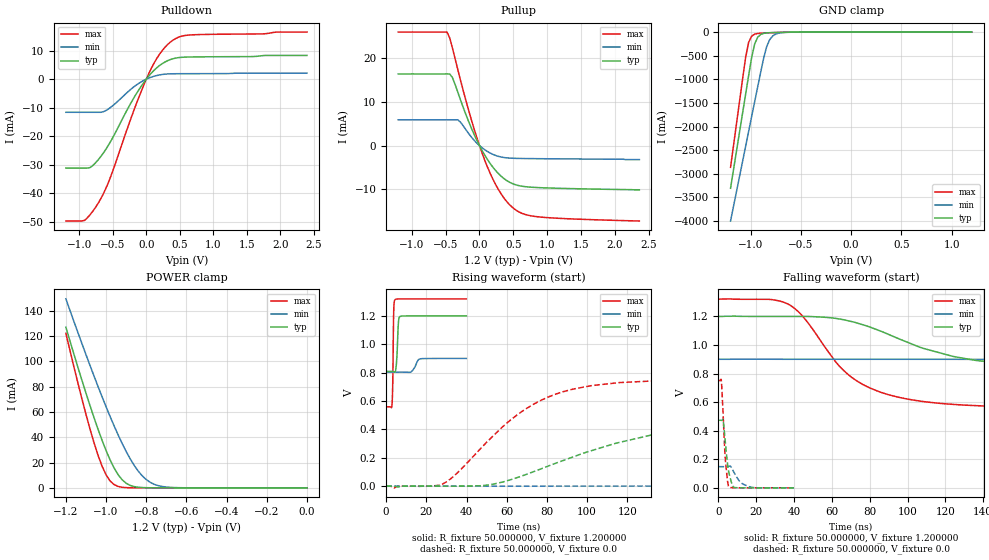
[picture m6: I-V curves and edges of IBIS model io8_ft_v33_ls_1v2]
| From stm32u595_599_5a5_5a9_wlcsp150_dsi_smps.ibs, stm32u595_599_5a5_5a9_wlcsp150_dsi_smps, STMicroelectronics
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|   Model io8_ft_v33_ls_1v2
[Model]  io8_ft_v33_ls_1v2
Model_type I/O
Polarity   Non-Inverting
Enable   Active-Low
Vinl =   0.360000V
Vinh =   0.840000V
Vmeas =  0.600000V
Cref =   50.000000pF
Rref =   100.000000M
Vref =   0.0V
C_comp   2.887200pF   2.816900pF   2.935200pF
[Temperature Range]   25.000000   0.140000k   -40.000000
[Pullup Reference]   1.200000V   0.900000V   1.320000V
[Pulldown Reference]   0.0V   0.0V   0.0V
[POWER Clamp Reference]   1.200000V   0.900000V   1.320000V
[GND Clamp Reference]   0.0V   0.0V   0.0V
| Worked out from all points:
|   slope of the pulldown table from 0 to 0.18 V, typ, clamps not added: 40.7 ohm
|   slope of the pullup table from 0 to 0.18 V, typ, clamps not added: 39.5 ohm
|   GND clamp passes 1 mA (typ) near -0.51 V on its own axis
|   POWER clamp passes 1 mA (typ) near -0.86 V on its own axis
|   rising waveform, R_fixture 50.000000, V_fixture 1.200000: 20-80 % time 752ps typ, 2.06ns min, 414ps max; typ from 0.809 V to 1.2 V
|   rising waveform, R_fixture 50.000000, V_fixture 0.0: 20-80 % time 67.6ns typ, 169ns min, 37.1ns max; typ from 0 V to 0.473 V
|   falling waveform, R_fixture 50.000000, V_fixture 1.200000: 20-80 % time 58.5ns typ, 150ns min, 31.6ns max; typ from 1.2 V to 0.809 V
|   falling waveform, R_fixture 50.000000, V_fixture 0.0: 20-80 % time 2.49ns typ, 4.76ns min, 1.84ns max; typ from 0.473 V to 0 V
[Pulldown]
|Voltage   I(typ)   I(min)   I(max)
-1.2V     -31.16mA   -11.61mA   -49.71mA
-920mV    -31.16mA   -11.61mA   -49.48mA
-840mV    -31mA      -11.61mA   -47.54mA
-720mV    -28.32mA   -11.61mA   -43.58mA
-560mV    -22.95mA   -10.37mA   -35.89mA
-200mV    -7.146mA   -2.964mA   -11.89mA
0V        0A         0A         0A
160mV     4.047mA    1.298mA    7.361mA
360mV     6.87mA     1.87mA     13mA
480mV     7.543mA    1.91mA     14.69mA
640mV     7.764mA    1.923mA    15.46mA
2.4V      8.316mA    2.102mA    16.52mA
[Pullup]
|Voltage   I(typ)   I(min)   I(max)
-1.2V     16.39mA    5.9mA      25.97mA
-480mV    16.39mA    5.9mA      25.97mA
-440mV    16.39mA    5.9mA      24.63mA
-400mV    15.57mA    5.9mA      22.35mA
-320mV    12.21mA    5.9mA      17.37mA
-120mV    3.997mA    1.962mA    5.905mA
80mV      -2.237mA   -962.6uA   -3.434mA
280mV     -6.404mA   -2.453mA   -10.06mA
520mV     -8.88mA    -2.901mA   -14.54mA
680mV     -9.389mA   -2.951mA   -15.76mA
920mV     -9.627mA   -2.991mA   -16.35mA
2.36V     -10.1mA    -3.2mA     -17.23mA
[GND_clamp]
|Voltage   I(typ)   I(min)   I(max)
-1.2V     -3.305A    -3.998A    -2.862A
-1.05V    -1.316A    -2.418A    -539.3mA
-1.02V    -921mA     -2.103A    -218.8mA
-990mV    -539.5mA   -1.788A    -87.43mA
-960mV    -252.1mA   -1.474A    -44.36mA
-930mV    -110.5mA   -1.16A     -30.32mA
-870mV    -28.03mA   -549.1mA   -21.09mA
-840mV    -18.43mA   -305.6mA   -18.27mA
-810mV    -13.9mA    -159.7mA   -15.73mA
-780mV    -11.23mA   -82.35mA   -13.37mA
-600mV    -2.976mA   -4.272mA   -3.058mA
1.2V      0A         14.74nA    0A
[POWER_clamp]
|Voltage   I(typ)   I(min)   I(max)
-1.2V     127mA      149.4mA    122.2mA
-1.12V    84.97mA    114mA      70.27mA
-1.06V    55.51mA    88.42mA    35.67mA
-1.02V    37.63mA    72.04mA    17.17mA
-1V       29.51mA    64.13mA    10.3mA
-960mV    15.69mA    48.99mA    2.571mA
-900mV    3.624mA    28.77mA    182.8uA
-840mV    490.7uA    13.24mA    11.35uA
-800mV    116.8uA    6.532mA    1.77uA
-740mV    13.2uA     1.723mA    109.1nA
-620mV    167.3nA    79.35uA    0A
0V        0A         17.84nA    0A
[Ramp]
| variable   typ   min   max
dV/dt_r  0.28374/67.55993n   88.87187m/0.16834u  0.45090/37.04554n
dV/dt_f  0.23463/58.41528n   57.86400m/0.14978u  0.45666/31.55745n
R_load = 50.000000
[Rising Waveform]
R_fixture= 50.000000
V_fixture= 1.200000
V_fixture_min= 0.900000
V_fixture_max= 1.320000
|time   V(typ)   V(min)   V(max)
0s        809mV      803.5mV    558.9mV
2.883ns   809.1mV    803.5mV    568.2mV
3.283ns   809mV      803.5mV    730.5mV
3.764ns   807.6mV    803.5mV    1.237V
4.404ns   804.5mV    803.5mV    1.314V
5.205ns   883.7mV    803.5mV    1.319V
6.166ns   1.164V     803.5mV    1.319V
6.807ns   1.195V     803.5mV    1.32V
16.98ns   1.2V       897.4mV    1.32V
39.88ns   1.2V       900mV      1.32V
[Rising Waveform]
R_fixture= 50.000000
V_fixture= 0.0
V_fixture_min= 0.0
V_fixture_max= 0.0
|time   V(typ)   V(min)   V(max)
0s        2.277nV    212.1nV    1.455nV
28.03ns   -71.47uV   -26.54uV   14mV
52.05ns   10.76mV    -20.37uV   337.8mV
74.07ns   105.7mV    7.748uV    583.1mV
92.09ns   201.2mV    73.5uV     680.8mV
118.1ns   315mV      425.6uV    731.4mV
168.2ns   427.6mV    6.838mV    749.9mV
244.2ns   467mV      48.53mV    751.6mV
452.5ns   472.9mV    134.9mV    751.5mV
997ns     472.9mV    148.2mV    751.6mV
[Falling Waveform]
R_fixture= 50.000000
V_fixture= 1.200000
V_fixture_min= 0.900000
V_fixture_max= 1.320000
|time   V(typ)   V(min)   V(max)
0s        1.2V       900mV      1.32V
36.04ns   1.2V       900mV      1.291V
44.04ns   1.2V       900mV      1.209V
64.06ns   1.182V     900mV      850.1mV
76.08ns   1.143V     900mV      725.6mV
98.1ns    1.029V     900mV      626.3mV
130.1ns   905.9mV    899.5mV    579.2mV
254.3ns   814.8mV    861.6mV    559mV
444.4ns   809.1mV    812.7mV    558.9mV
997ns     809mV      803.5mV    558.9mV
[Falling Waveform]
R_fixture= 50.000000
V_fixture= 0.0
V_fixture_min= 0.0
V_fixture_max= 0.0
|time   V(typ)   V(min)   V(max)
0s        472.9mV    148.2mV    751.6mV
1.522ns   472.6mV    148.2mV    750.4mV
2.482ns   473.4mV    148.2mV    504.1mV
3.604ns   321.3mV    148.2mV    203.9mV
4.885ns   157.2mV    148.1mV    38.86mV
5.606ns   99.79mV    150.3mV    4.93mV
8.088ns   3.599mV    111mV      626uV
11.61ns   435.7uV    39.56mV    38.94uV
16.02ns   30.58uV    9.023mV    -21.61uV
39.88ns   2.277nV    212.1nV    1.455nV
